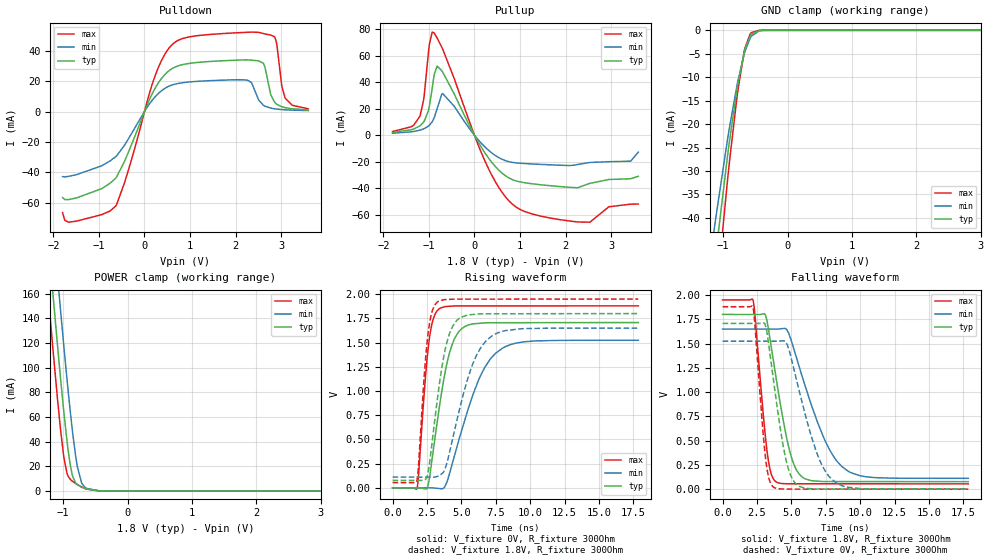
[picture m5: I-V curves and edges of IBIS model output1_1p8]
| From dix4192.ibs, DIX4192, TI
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|   output1_1p8 Model
[Model]   output1_1p8
Model_type   3-state
Polarity   Non-Inverting
Vmeas = 0.9
Vref = 0
Cref = 2pF
Rref = 100000
|   typ   min   max
C_comp   31.1631pF   25.2142pF   36.9522pF
|C_comp_pullup   31.7419pF   25.9188pF   37.6389pF
|C_comp_pulldown   31.5947pF   25.8012pF   37.4646pF
| Where nom  PVT is Nominal Process, 1.8V, 27C
|   Fast PVT is Strong Process,  1.95V, -40C
|   Slow PVT is Weak Process,   1.65V, 105C
[Voltage Range]   1.8   1.65   1.95
[Temperature Range]   27   105   -40
[Pullup Reference]   1.8   1.65   1.95
[Pulldown Reference]   0   0   0
[Power Clamp Reference]   1.8   1.65   1.95
[GND Clamp Reference]   0   0   0
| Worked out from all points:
|   slope of the pulldown table from 0 to 0.27 V, typ, clamps not added: 15.7 ohm
|   slope of the pullup table from 0 to 0.27 V, typ, clamps not added: 17.7 ohm
|   GND clamp passes 1 mA (typ) near -0.57 V on its own axis
|   POWER clamp passes 1 mA (typ) near -0.56 V on its own axis
|   falling waveform, V_fixture 1.8V, R_fixture 300Ohm: 20-80 % time 1.28ns typ, 2.33ns min, 715ps max; typ from 1.8 V to 0.077 V
|   rising waveform, V_fixture 0V, R_fixture 300Ohm: 20-80 % time 1.17ns typ, 2.16ns min, 634ps max; typ from 0 V to 1.71 V
|   rising waveform, V_fixture 1.8V, R_fixture 300Ohm: 20-80 % time 1.04ns typ, 1.79ns min, 585ps max; typ from 0.077 V to 1.8 V
|   falling waveform, V_fixture 0V, R_fixture 300Ohm: 20-80 % time 1.08ns typ, 1.83ns min, 632ps max; typ from 1.71 V to 0 V
[Pulldown]
|   Voltage   I(typ)   I(min)   I(max)
-1.8V     -56.63mA   -42.82mA   -66.47mA
-1.67V    -57.96mA   -42.69mA   -72.85mA
-633.6mV  -43.89mA   -29.74mA   -62.3mA
273.6mV   17.4mA     10.99mA    26.7mA
765mV     30.33mA    18.63mA    47.27mA
2.266V    34.03mA    20.63mA    52.22mA
2.509V    33.35mA    7.565mA    52.15mA
2.617V    31.56mA    4.064mA    51.33mA
2.855V    6.344mA    1.84mA     49.25mA
3.017V    3.179mA    1.318mA    16.68mA
3.087V    2.59mA     1.171mA    9.115mA
3.6V      1.075mA    640.9uA    1.804mA
[GND Clamp]
|   Voltage   I(typ)   I(min)   I(max)
-1.8V     -142.4mA   -115.4mA   -175.1mA
-1.174V   -55.01mA   -45.84mA   -66.67mA
-1.114V   -47.68mA   -39.97mA   -57.72mA
-930.6mV  -26.64mA   -23.12mA   -31.76mA
-898.2mV  -23.26mA   -20.41mA   -27.55mA
-784.8mV  -12.59mA   -11.75mA   -14.21mA
-671.4mV  -4.573mA   -4.985mA   -4.394mA
-579.6mV  -1.113mA   -1.637mA   -749.3uA
-563.4mV  -804.9uA   -1.274mA   -497.5uA
-444.6mV  -42.08uA   -128uA     -11.6uA
-347.4mV  -1.97uA    -12.75uA   -90.19nA
3.6V      0A         0A         0A
[Pullup]
|   Voltage   I(typ)   I(min)   I(max)
-1.8V     2.198mA    1.55mA     2.867mA
-1.201V   7.084mA    3.863mA    14.25mA
-1.114V   10.13mA    4.875mA    27.64mA
-1.017V   18.04mA    6.818mA    60.52mA
-925.2mV  36.38mA    10.47mA    77.67mA
-822.6mV  51.95mA    19.8mA     73.34mA
-698.4mV  47.53mA    31.43mA    64.82mA
235.8mV   -13.6mA    -8.983mA   -19.78mA
840.6mV   -33.45mA   -20.44mA   -52.05mA
2.536V    -36.15mA   -20.44mA   -65.37mA
2.952V    -33.25mA   -19.84mA   -53.78mA
3.6V      -30.84mA   -12.63mA   -51.67mA
[POWER Clamp]
|   Voltage   I(typ)   I(min)   I(max)
-1.8V     564.8mA    620.9mA    520.8mA
-1.233V   204.8mA    261.9mA    159.6mA
-1.168V   165.5mA    222.3mA    120.5mA
-1.087V   117.7mA    173.8mA    74.13mA
-1.039V   90.27mA    145.4mA    48.83mA
-984.6mV  61.6mA     114.7mA    25.82mA
-941.4mV  40.98mA    91.12mA    14.65mA
-887.4mV  20.49mA    63.43mA    9.326mA
-806.4mV  6.463mA    28.45mA    6.043mA
-714.6mV  3.048mA    6.727mA    3.292mA
-412.2mV  29.87uA    75.2uA     8.813uA
3.6V      0A         0A         0A
[Ramp]
R_load = 300
|   typ   min   max
dV/dt_r   1.02457/1.17105e-09   0.914683/2.16305e-09   1.12794/6.33929e-10
dV/dt_f   1.03368/1.27738e-09   0.923161/2.32907e-09   1.13713/7.1319e-10
[Falling Waveform]
V_fixture = 1.8V
V_fixture_min = 1.65V
V_fixture_max = 1.95V
R_fixture = 300Ohm
C_fixture = 0F
|   Time   V(typ)   V(min)   V(max)
0s        1.8V       1.65V      1.95V
2.212ns   1.8V       1.65V      1.947V
3.227ns   1.734V     1.65V      397mV
3.512ns   1.49V      1.65V      169.6mV
3.891ns   1.144V     1.65V      75.18mV
4.658ns   527.6mV    1.645V     56mV
5.414ns   187.5mV    1.335V     55.25mV
7.34ns    78.85mV    534.3mV    55.18mV
8.647ns   78.64mV    235.8mV    55.13mV
17.86ns   77.2mV     111.4mV    54.79mV
[Rising Waveform]
V_fixture = 0V
V_fixture_min = 0V
V_fixture_max = 0V
R_fixture = 300Ohm
C_fixture = 0F
|   Time   V(typ)   V(min)   V(max)
0s        -524.7nV   1.516uV    -30.53nV
1.783ns   107.6uV    88.21uV    -717.8uV
2.621ns   53.58mV    129uV      1.483V
2.929ns   357mV      -530.7uV   1.731V
3.386ns   821.8mV    -6.884mV   1.849V
4.032ns   1.337V     96.45mV    1.874V
4.777ns   1.607V     474.2mV    1.879V
6.436ns   1.701V     1.172V     1.879V
7.986ns   1.706V     1.443V     1.879V
17.86ns   1.708V     1.524V     1.88V
[Rising Waveform]
V_fixture = 1.8V
V_fixture_min = 1.65V
V_fixture_max = 1.95V
R_fixture = 300Ohm
C_fixture = 0F
|   Time   V(typ)   V(min)   V(max)
0s        77.2mV     111.4mV    54.79mV
1.767ns   76.85mV    111.1mV    72.82mV
2.555ns   141.5mV    111mV      1.564V
2.87ns    468.9mV    110.9mV    1.819V
3.286ns   947.5mV    119.7mV    1.922V
3.899ns   1.476V     233.6mV    1.945V
4.527ns   1.705V     607.1mV    1.949V
5.872ns   1.791V     1.296V     1.949V
7.264ns   1.798V     1.574V     1.949V
17.86ns   1.8V       1.65V      1.95V
[Falling Waveform]
|Gnd
V_fixture = 0V
V_fixture_min = 0V
V_fixture_max = 0V
R_fixture = 300Ohm
C_fixture = 0F
|   Time   V(typ)   V(min)   V(max)
0s        1.708V     1.524V     1.88V
2.212ns   1.707V     1.524V     1.872V
3.108ns   1.689V     1.524V     339.4mV
3.363ns   1.48V      1.524V     114.2mV
3.689ns   1.134V     1.524V     22.36mV
4.527ns   356.6mV    1.524V     554.9uV
5.194ns   77.44mV    1.23V      458.6uV
6.848ns   1.383mV    373.5mV    398.7uV
8.278ns   1.203mV    63.76mV    346.9uV
17.86ns   -520.4nV   1.516uV    -25.43nV
